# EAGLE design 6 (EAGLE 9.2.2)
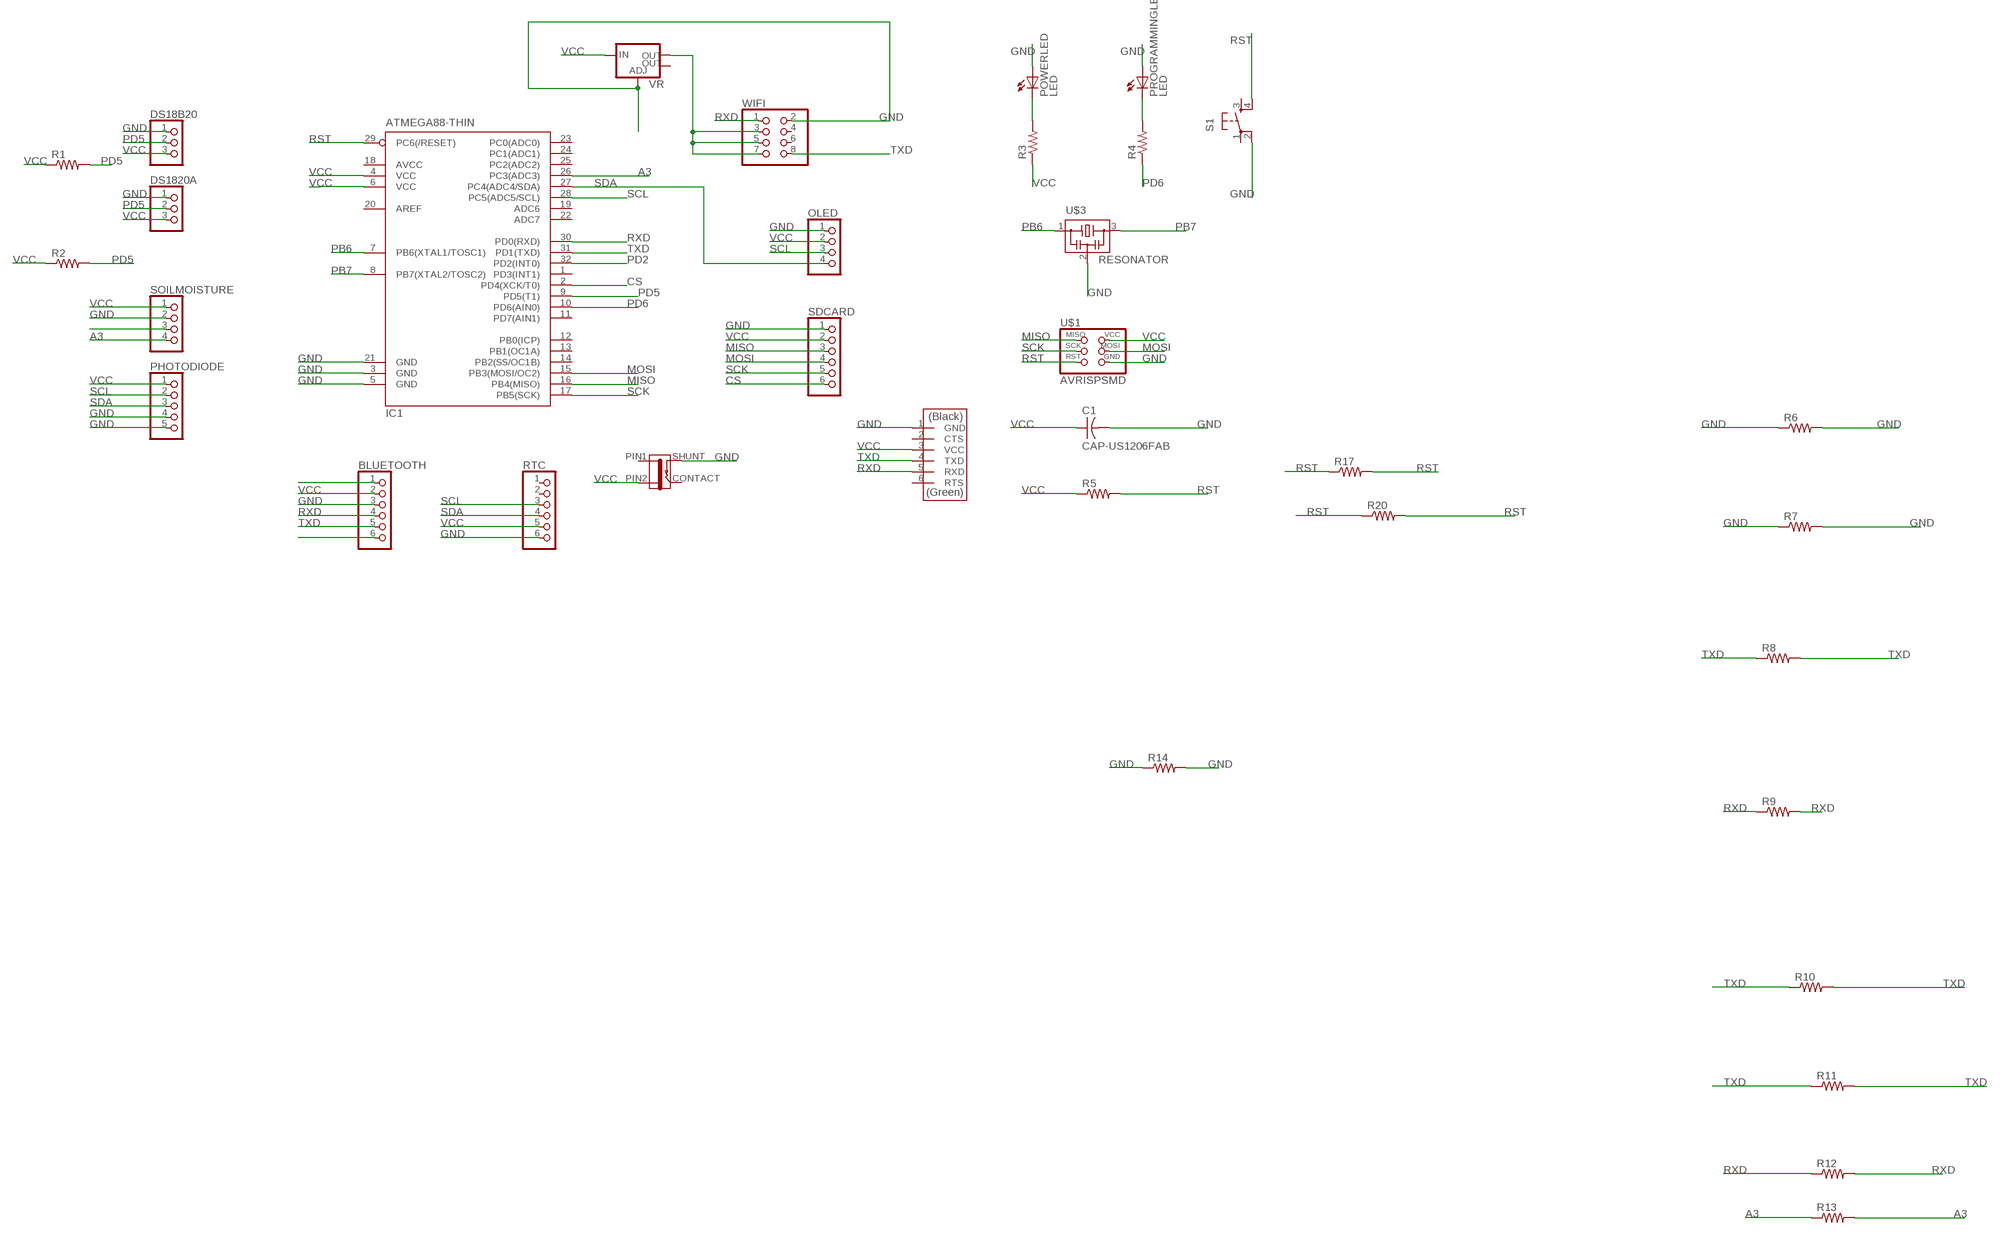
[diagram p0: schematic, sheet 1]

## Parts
BLUETOOTH  PINHD-1X6  [1X06]
C1  CAP-US1206FAB  [C1206FAB]
DS18B20  PINHD-1X3  [1X03]
DS1820A  PINHD-1X3  [1X03]
FTDI  FTDI-SMD-HEADER  [1X06SMD]
IC1  ATMEGA88-THIN  [TQFP32-08THIN]
J1  JACK-2.1MM  [PJ-002AH-SMT]
OLED  PINHD-1X4  [1X04]
PHOTODIODE  PINHD-1X5  [1X05]
POWERLED  LED  [LED1206]
PROGRAMMINGLED  LED  [LED1206]
R1  RES-US1206FAB  [R1206FAB]
R2  RES-US1206FAB  [R1206FAB]
R3  RES-US1206FAB  [R1206FAB]
R4  RES-US1206FAB  [R1206FAB]
R5  RES-US1206FAB  [R1206FAB]
R6  RES-US1206FAB  [R1206FAB]
R7  RES-US1206FAB  [R1206FAB]
R8  RES-US1206FAB  [R1206FAB]
R9  RES-US1206FAB  [R1206FAB]
R10  RES-US1206FAB  [R1206FAB]
R11  RES-US1206FAB  [R1206FAB]
R12  RES-US1206FAB  [R1206FAB]
R13  RES-US1206FAB  [R1206FAB]
R14  RES-US1206FAB  [R1206FAB]
R17  RES-US1206FAB  [R1206FAB]
R20  RES-US1206FAB  [R1206FAB]
RTC  PINHD-1X6  [1X06]
S1  6MM_SWITCH6MM_SWITCH  [6MM_SWITCH]
SDCARD  PINHD-1X6  [1X06]
SOILMOISTURE  PINHD-1X4  [1X04]
U$1  AVRISPSMD  [2X03SMD]
U$3  RESONATOR  [EFOBM]
VR  V_REG_LM1117SOT223  [SOT223]
WIFI  PINHD-2X4  [2X04]

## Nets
A3: IC1.26(PC3(ADC3)) R13.1 R13.2 SOILMOISTURE.4
CS: IC1.2(PD4(XCK/T0)) SDCARD.6
GND: BLUETOOTH.3 C1.2 DS18B20.1 DS1820A.1 FTDI.1(GND) IC1.3(GND) IC1.5(GND) IC1.21(GND) J1.SHUNT OLED.1 PHOTODIODE.4 PHOTODIODE.5 POWERLED.1(A) PROGRAMMINGLED.1(A) R6.1 R6.2 R7.1 R7.2 R14.1 R14.2 RTC.6 S1.2(P1) SDCARD.1 SOILMOISTURE.2 U$1.6(GND) U$3.2 VR.1(ADJ) WIFI.2
MISO: IC1.16(PB4(MISO)) SDCARD.3 U$1.1(MISO)
MOSI: IC1.15(PB3(MOSI/OC2)) SDCARD.4 U$1.4(MOSI)
N$1: BLUETOOTH.1
N$2: VR.2(OUT) WIFI.3 WIFI.5 WIFI.7
N$4: SOILMOISTURE.3
N$6: POWERLED.2(C) R3.2
N$8: BLUETOOTH.6
N$10: PROGRAMMINGLED.2(C) R4.2
PB6: IC1.7(PB6(XTAL1/TOSC1)) U$3.1
PB7: IC1.8(PB7(XTAL2/TOSC2)) U$3.3
PD2: IC1.32(PD2(INT0))
PD5: DS18B20.2 DS1820A.2 IC1.9(PD5(T1)) R1.2 R2.2
PD6: IC1.10(PD6(AIN0)) R4.1
RST: IC1.29(PC6(/RESET)) R5.2 R17.1 R17.2 R20.1 R20.2 S1.4(S1) U$1.5(RST)
RXD: BLUETOOTH.4 FTDI.5(RXD) IC1.30(PD0(RXD)) R9.1 R9.2 R12.1 R12.2 WIFI.1
SCK: IC1.17(PB5(SCK)) SDCARD.5 U$1.3(SCK)
SCL: IC1.28(PC5(ADC5/SCL)) OLED.3 PHOTODIODE.2 RTC.3
SDA: IC1.27(PC4(ADC4/SDA)) OLED.4 PHOTODIODE.3 RTC.4
TXD: BLUETOOTH.5 FTDI.4(TXD) IC1.31(PD1(TXD)) R8.1 R8.2 R10.1 R10.2 R11.1 R11.2 WIFI.8
VCC: BLUETOOTH.2 C1.1 DS18B20.3 DS1820A.3 FTDI.3(VCC) IC1.4(VCC) IC1.6(VCC) J1.PIN2 OLED.2 PHOTODIODE.1 R1.1 R2.1 R3.1 R5.1 RTC.5 SDCARD.2 SOILMOISTURE.1 U$1.2(VCC) VR.3(IN)
Unconnected: FTDI.2(CTS) FTDI.6(RTS) IC1.1(PD3(INT1)) IC1.11(PD7(AIN1)) IC1.12(PB0(ICP)) IC1.13(PB1(OC1A)) IC1.14(PB2(SS/OC1B)) IC1.19(ADC6) IC1.20(AREF) IC1.22(ADC7) IC1.23(PC0(ADC0)) IC1.24(PC1(ADC1)) IC1.25(PC2(ADC2)) RTC.1 RTC.2 S1.1(P) S1.3(S) VR.4(OUT) WIFI.4 WIFI.6

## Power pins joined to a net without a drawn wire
AVCC: IC1.18(AVCC)
CONTACT: J1.CONTACT
PIN1: J1.PIN1

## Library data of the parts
BLUETOOTH RTC SDCARD = pinhead:PINHD-1X6: PIN HEADER
C1 = fab:CAP-US
DS18B20 DS1820A = pinhead:PINHD-1X3: PIN HEADER
FTDI = fab:FTDI-SMD-HEADER
IC1 = fab:ATMEGA88-THIN
J1 = fab:JACK-2.1MM: SMD DC power jack PJ-002AH-SMT As found in the fablab inventory. Made by Zaerc.
OLED SOILMOISTURE = pinhead:PINHD-1X4: PIN HEADER
PHOTODIODE = pinhead:PINHD-1X5: PIN HEADER
POWERLED PROGRAMMINGLED = fab:LED: LED
R1-R14 R17 R20 = fab:RES-US: Resistor (US Symbol)
S1 = fab:6MM_SWITCH: OMRON SWITCH
U$1 = fab:AVRISP
U$3 = fab:RESONATOR
VR = fab:V_REG_LM1117: Voltage Regulator LM1117 Standard adjustable voltage regulator but in SMD form. Spark Fun Electronics SKU : COM-00595; PROD_ID: VREG-08170
WIFI = pinhead:PINHD-2X4: PIN HEADER

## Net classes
0 default: width 0.152 mm, clearance 0.4 mm

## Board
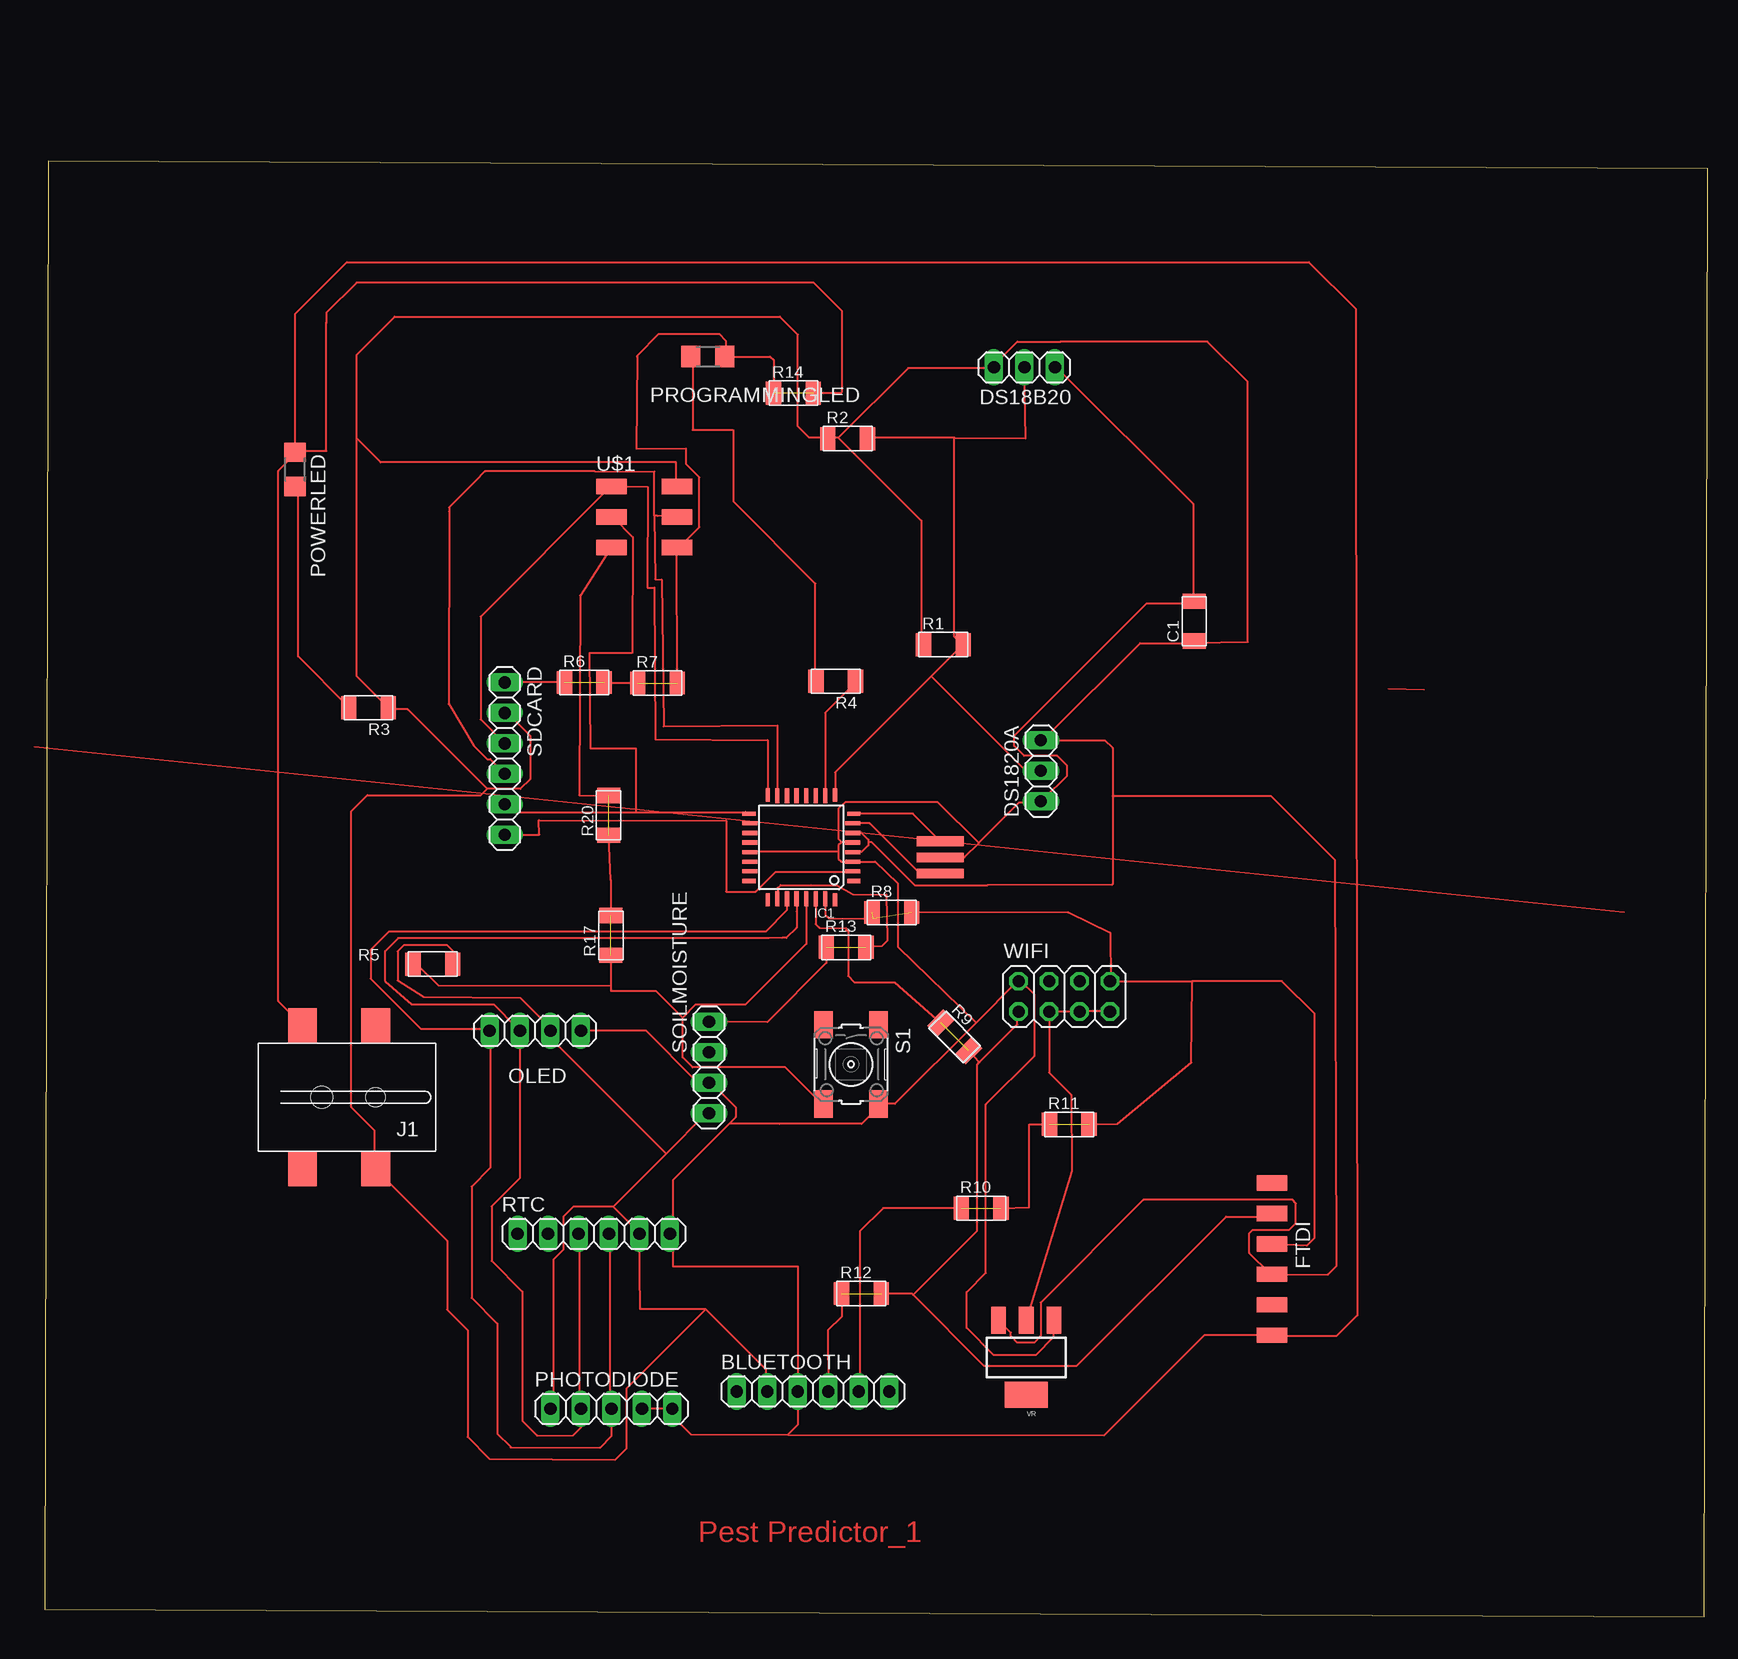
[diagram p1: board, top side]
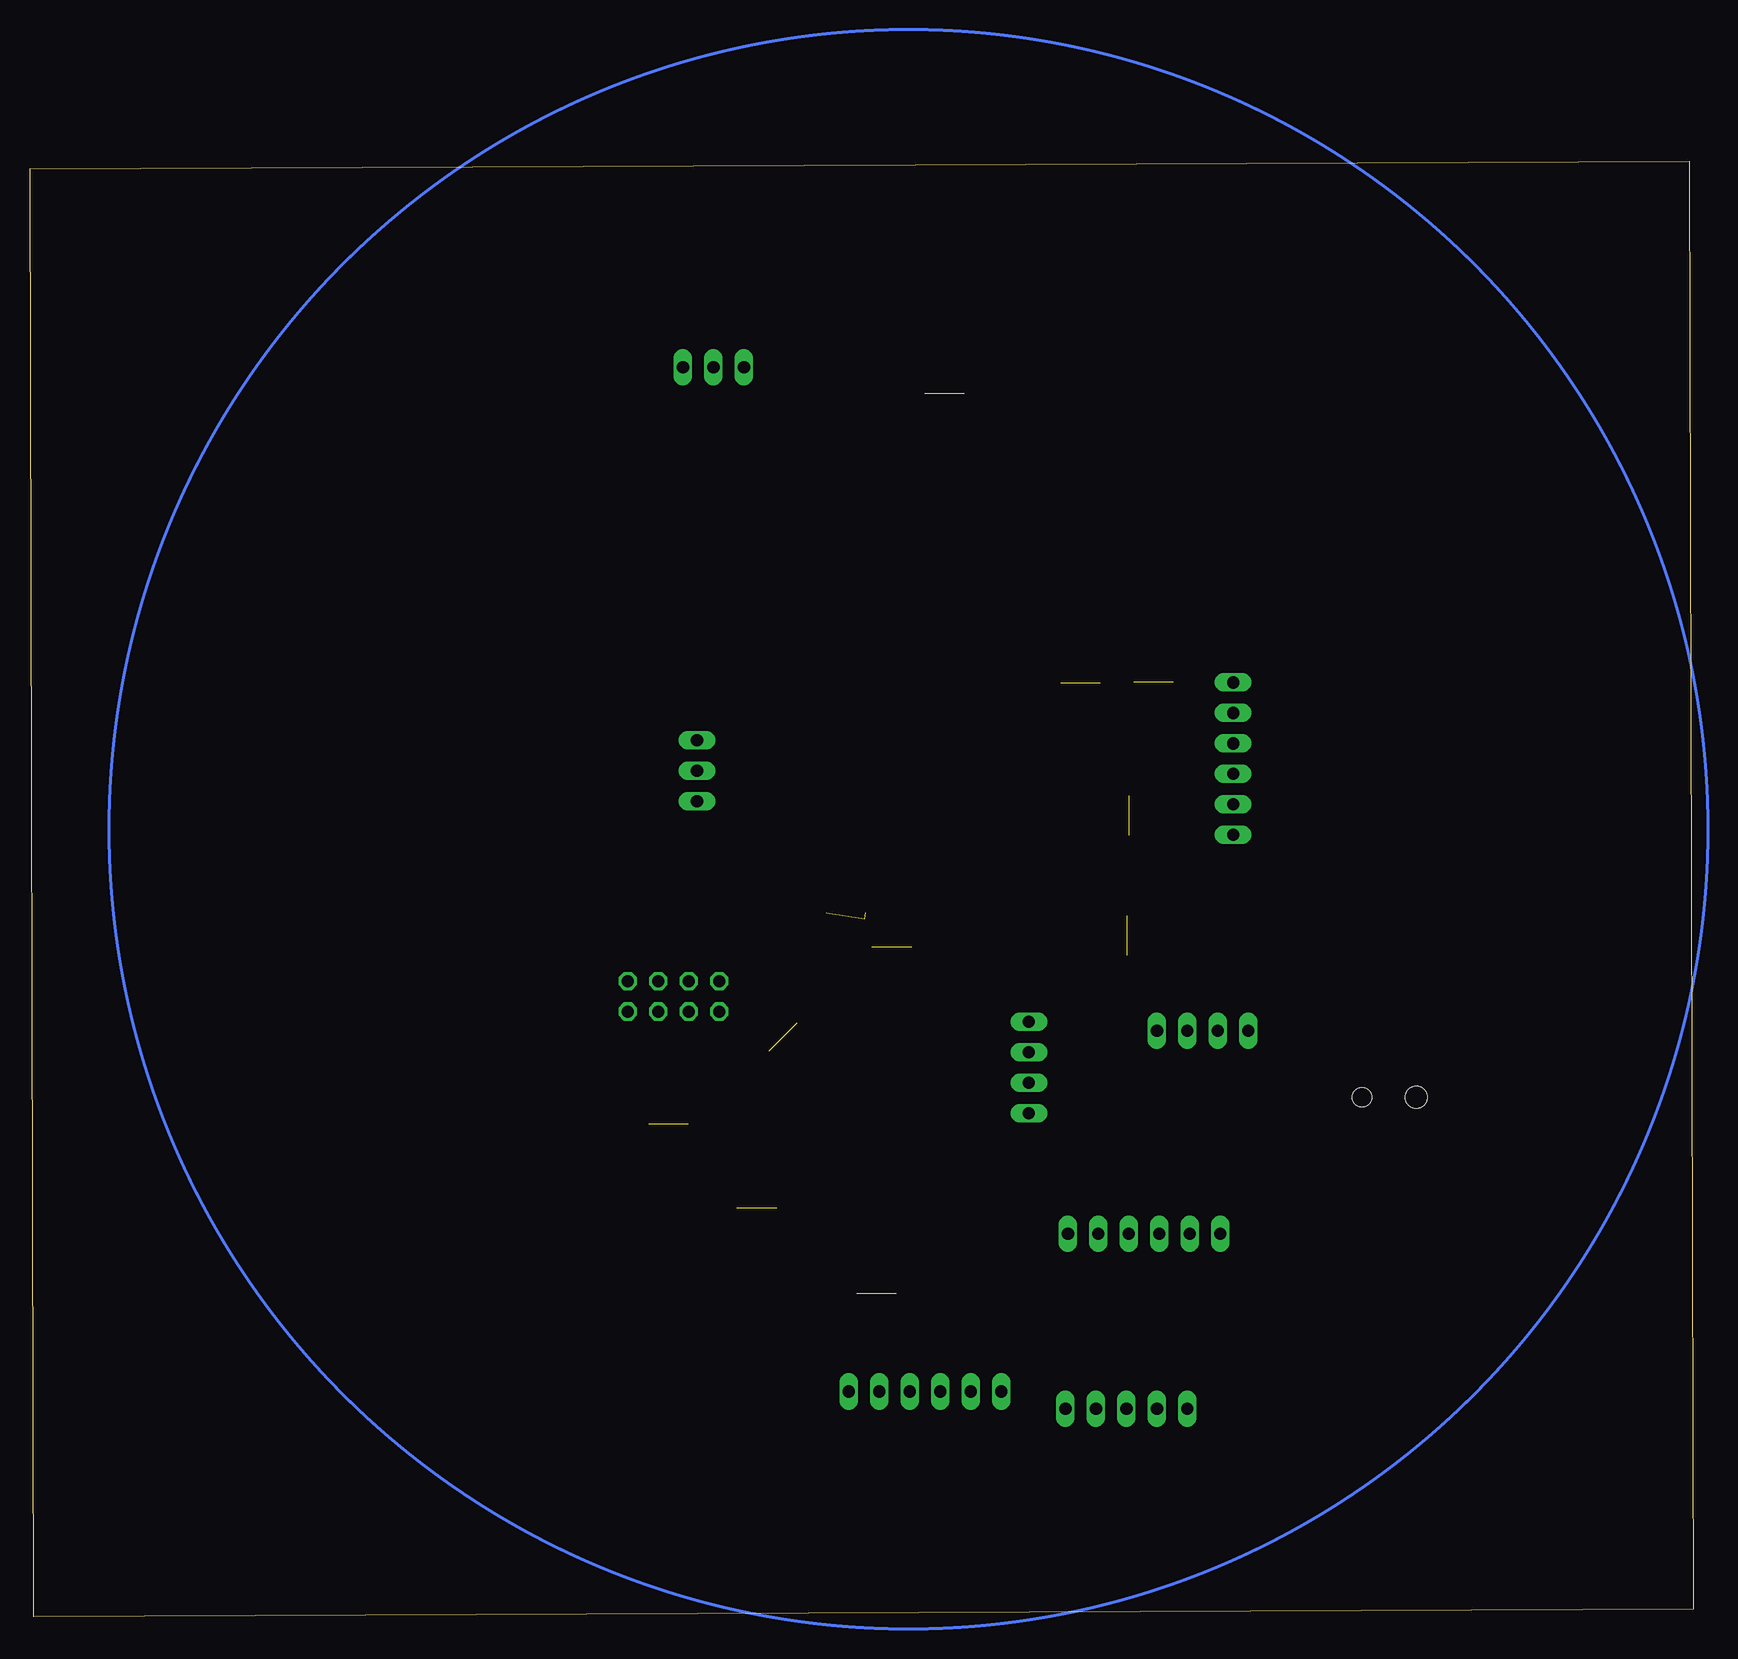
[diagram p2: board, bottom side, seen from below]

Size 138.59 x 121.29 mm. Coordinates in mm from the lower left corner, seen from the top.
Outline: 0,0.61 138.28,0 138.59,120.68 0.3,121.29 0,0.61
Copper layers (1*16): Top 0.035mm / dielectric 1.5mm / Bottom 0.035mm
Design rules "default *": minimum track width 6mil, minimum drill 0.35mm, track to track 0.4mm, track to pad 6mil, pad to pad 6mil, via to via 6mil, smd to smd 6mil, copper to edge 40mil, drill to drill 6mil, minimum pad ring 10mil, minimum via ring 8mil, stop-mask expansion 4mil, vias tented up to drill 0mil, thermal gap 10mil

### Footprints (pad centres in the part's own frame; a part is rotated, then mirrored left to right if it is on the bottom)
1X06 = drill 1.016 long: 1 -6.35,0; 2 -3.81,0; 3 -1.27,0; 4 1.27,0; 5 3.81,0; 6 6.35,0
C1206FAB = smd 1.27 x 1.905: 1 -1.651,0; 2 1.651,0
1X03 = drill 1.016 long: 1 -2.54,0; 2 0,0; 3 2.54,0
1X06SMD = smd 2.54 x 1.27: 1 0,6.35; 2 0,3.81; 3 0,1.27; 4 0,-1.27; 5 0,-3.81; 6 0,-6.35
TQFP32-08THIN = smd 1.118 x 0.356: 1 -4.369,2.8; 8 -4.369,-2.8; 17 4.369,-2.8; 24 4.369,2.8 | smd 1.27 x 0.356: 2 -4.293,2; 3 -4.293,1.2; 4 -4.293,0.4; 5 -4.293,-0.4; 6 -4.293,-1.2; 7 -4.293,-2; 18 4.293,-2; 19 4.293,-1.2; 20 4.293,-0.4; 21 4.293,0.4; 22 4.293,1.2; 23 4.293,2 | smd 0.356 x 1.118: 9 -2.8,-4.369; 16 2.8,-4.369; 25 2.8,4.369; 32 -2.8,4.369 | smd 0.356 x 1.27: 10 -2,-4.293; 14 1.2,-4.293; 15 2,-4.293; 26 2,4.293; 27 1.2,4.293; 31 -2,4.293 | smd 0.35 x 1.27: 11 -1.2,-4.293; 12 -0.4,-4.293; 13 0.4,-4.293; 28 0.4,4.293; 29 -0.4,4.293; 30 -1.2,4.293
PJ-002AH-SMT = smd 2.4 x 2.8: CONTACT -2.4,-6; PIN1 3.7,6; PIN2 -2.4,6; SHUNT 3.7,-6 | hole 1.6: -2.4,0 | hole 1.8: 2.1,0
1X04 = drill 1.016 long: 1 -3.81,0; 2 -1.27,0; 3 1.27,0; 4 3.81,0
1X05 = drill 1.016 long: 1 -5.08,0; 2 -2.54,0; 3 0,0; 4 2.54,0; 5 5.08,0
LED1206 = smd 1.6 x 1.803: 1 -1.422,0; 2 1.422,0
R1206FAB = smd 1.27 x 1.905: 1 -1.651,0; 2 1.651,0
6MM_SWITCH = smd 2.286 x 1.524: 1 -3.302,2.286; 2 3.302,2.286; 3 -3.302,-2.286; 4 3.302,-2.286
2X03SMD = smd 2.54 x 1.27: 1 -2.54,2.54; 2 2.92,2.54; 3 -2.54,0; 4 2.92,0; 5 -2.54,-2.54; 6 2.92,-2.54
EFOBM = smd 0.8 x 3.9: 1 -1.35,0; 2 0,0; 3 1.35,0
SOT223 = smd 1.219 x 2.235: 1 -2.311,-3.099; 2 0,-3.099; 3 2.311,-3.099 | smd 3.6 x 2.2: 4 0,3.099
2X04 = drill 1.016 octagon: 1 -3.81,-1.27; 2 -3.81,1.27; 3 -1.27,-1.27; 4 -1.27,1.27; 5 1.27,-1.27; 6 1.27,1.27; 7 3.81,-1.27; 8 3.81,1.27

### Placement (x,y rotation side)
BLUETOOTH  64.01,18.77 0 top
C1  95.78,82.96 90 top
DS18B20  81.64,104.11 180 top
DS1820A  83.01,70.48 90 top
FTDI  102.29,29.79 180 top
IC1  63.04,64.11 180 top
J1  25.17,43.28 180 top
OLED  40.87,48.82 180 top
PHOTODIODE  47.22,17.32 0 top
POWERLED  20.85,95.61 270 top
PROGRAMMINGLED  55.24,105 180 top
R1  74.88,81 0 top
R2  66.9,98.17 0 top
R3  26.97,75.74 180 top
R4  65.91,77.95 180 top
R5  32.33,54.38 180 top
R6  44.96,77.85 0 top
R7  51.05,77.8 0 top
R8  70.59,58.67 0 top
R9  75.82,48.31 315 top
R10  78.03,34.04 0 top
R11  85.37,41.02 0 top
R12  68.05,26.92 0 top
R13  66.78,55.78 0 top
R14  62.38,101.96 0 top
R17  47.17,56.77 90 top
R20  46.99,66.78 90 top
RTC  45.75,31.9 0 top
S1  67.18,46.02 270 top
SDCARD  38.33,71.5 270 top
SOILMOISTURE  55.35,45.77 90 top
U$1  49.76,91.64 0 top
U$3  74.63,63.27 90 top
VR  81.79,21.59 180 top
WIFI  84.96,51.69 0 top

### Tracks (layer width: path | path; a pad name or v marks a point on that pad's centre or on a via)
A3  (1 unrouted)
  Top 0.152: IC1.26 61.07,59.83 61.07,60.71 61.32,60.96 63.83,60.96 65.99,60.96 67.34,60.2 70.13,60.17 70.22,56.46 70.22,56.34 69.75,55.87 R13.2 | SOILMOISTURE.4 60.2,49.55 65.13,54.48 R13.1
CS
  Top 0.152: IC1.2 67.24,62.07 60.89,62.07 59.24,60.41 56.77,60.41 56.77,66.35 41.17,66.37 41.22,65.18 SDCARD.6
GND  (3 unrouted)
  Top 0.152: DS18B20.1 84.37,104.05 95.69,92.73 95.69,84.72 C1.2 95.69,84.44 91.83,84.44 80.78,73.39 80.78,72.56 81.61,71.73 84.37,71.73 85.2,70.91 85.2,70.08 83.26,68.14 DS1820A.1 82.99,67.87 81.21,67.87 77.82,64.48 | 66.14,63.72 66.14,64.28 66.42,64.55 | 66.14,63.72 66.14,63.17 66.42,62.9 67.24,62.9 IC1.3 | 66.42,64.55 67.24,64.55 IC1.5 | 66.14,63.72 58.96,63.72 IC1.21 | U$3.2 76.64,63.27 77.83,64.46 77.82,64.48 | 66.42,64.55 66.14,64.83 66.14,67.31 66.69,67.87 74.43,67.87 77.82,64.48 | 57.02,41.07 57.58,41.63 57.58,42.46 55.37,44.67 SOILMOISTURE.2 55.09,44.67 54.26,44.67 50.12,48.81 44.87,48.81 OLED.1 | 57.02,41.07 52.33,36.38 52.33,31.96 RTC.6 52.33,31.69 52.33,29.2 62.76,29.18 BLUETOOTH.3 62.74,15.99 61.92,15.18 | VR.1 84.09,24.5 84.09,23.32 82.56,21.79 79.09,21.79 76.81,24.07 76.81,27.04 78.42,28.65 78.42,42.7 82.44,46.71 82.44,51.85 81.33,52.95 WIFI.2 81.05,52.95 77.61,49.51 | 77.61,49.51 70.84,42.73 69.73,42.73 S1.2 69.45,42.46 68.07,41.08 61.21,41.08 61.22,41.07 57.02,41.07 | 67.52,62.9 IC1.3 | POWERLED.1 20.84,96.87 19.46,95.49 19.46,51.3 21.4,49.36 J1.SHUNT | PHOTODIODE.4 49.84,17.32 52.05,17.32 PHOTODIODE.5 | 102.05,23.4 FTDI.1 | 52.33,17.32 PHOTODIODE.5 | POWERLED.1 21.12,97.14 23.47,97.14 23.47,107.82 23.47,107.87 23.47,108.66 25.98,111.18 64.06,111.18 66.4,108.84 66.4,102.03 66.32,101.96 R14.2 | 102.32,23.4 FTDI.1 | 56.47,105.15 PROGRAMMINGLED.1 | R6.1 SDCARD.1 | R7.1 46.68,77.78 R6.2 | R7.2 U$1.6 52.69,89.11 52.8,89.12 52.88,89.13 54.54,90.79 54.54,94.93 53.43,96.04 53.43,97.36 49.3,97.33 49.36,104.95 49.36,105.08 51.18,106.89 56.18,106.89 56.74,106.34 56.74,105.06 56.8,105 PROGRAMMINGLED.1
  Top 0.152: IC1.3 69.19,62.92 71.09,61.11 71.09,55.83 77.61,49.51 | 61.92,15.18 53.85,15.19 52.3,16.74 PHOTODIODE.5 | 61.92,15.18 88.29,15.13 96.6,23.44 FTDI.1 | FTDI.1 102.34,23.39 107.65,23.39 109.35,25.1 109.39,25.1 109.28,101.14 109.28,108.93 105.33,112.88 25.17,112.88 20.85,108.56 POWERLED.1 | PROGRAMMINGLED.1 60.45,105 60.73,104.72 R14.1
MISO
  Top 0.152: IC1.16 60.24,73.05 50.88,73.1 50.8,85.75 50.22,85.75 50.24,94.16 U$1.1 47.08,94.11 36.31,83.33 36.31,74.77 38.24,72.84 SDCARD.3
MOSI
  Top 0.152: IC1.15 61.04,74.27 51.56,74.19 51.41,86.41 50.85,86.46 50.8,91.75 | SDCARD.4 38.24,70.35 37.14,71.46 36.86,71.46 35.76,72.56 33.65,76.07 33.7,92.1 33.7,92.45 35.91,94.67 36.68,95.43 45.85,95.44 50.8,95.43 50.8,91.75 | U$1.4 51.05,91.73 50.8,91.75
N$2
  Top 0.152: WIFI.7 88.51,50.47 86.3,50.47 WIFI.5 86.03,50.47 83.82,50.47 WIFI.3 83.69,45.33 85.56,43.46 85.52,43.46 85.58,37.14 VR.2
N$6
  Top 0.152: POWERLED.2 21.12,94.11 21.12,80.02 25.26,75.88 R3.2
N$10
  Top 0.152: PROGRAMMINGLED.2 53.99,104.88 53.99,98.91 57.35,98.91 57.37,92.93 64.21,86.1 64.21,78.09 R4.2
PB6
  Top 0.152: IC1.7 68.73,66.11 72.77,62.07 74.43,62.07 U$3.1
PB7
  Top 0.152: IC1.8 72.34,66.91 74.43,64.83 U$3.3
PD5
  Top 0.152: 75.81,98.25 68.63,98.25 R2.2 | 73.87,78.36 76.36,80.85 R1.2 76.36,81.12 75.81,81.68 75.81,98.25 | 73.87,78.36 65.86,70.35 65.86,68.7 IC1.9 | 73.87,78.36 81.61,70.63 82.99,70.63 DS1820A.2 | 75.81,98.25 81.74,98.2 DS18B20.2
PD6
  Top 0.152: IC1.10 65.04,68.42 65.04,75.32 67.52,77.81 R4.1
RST  (2 unrouted)
  Top 0.152: IC1.29 63.45,56.07 58.41,51.02 54.26,51.02 53.16,49.91 | 53.16,49.91 53.16,46.6 53.99,45.77 61.72,45.77 64.76,42.73 S1.4 | 53.16,49.91 50.95,52.12 47.17,52.12 47.17,52.58 | R5.2 30.79,54.33 31.06,54.33 32.79,52.6 47.17,52.58 | 47.34,88.98 U$1.5 44.6,85.08 44.52,68.45 R20.2 | R17.2 47.17,61.38 R20.1 | R17.1 47.17,52.58
RXD  (2 unrouted)
  Top 0.152: FTDI.5 102.05,33.34 98.44,33.34 86.01,20.91 78.26,20.91 72.36,26.81 | 77.89,46.19 77.69,46 77.69,32.15 72.36,26.81 | 77.89,46.19 81.05,49.36 81.05,50.19 WIFI.1 | 77.89,46.19 R9.2 | BLUETOOTH.4 65.26,23.85 66.4,24.98 R12.1 | R9.1 70.82,52.86 67.47,52.86 66.93,53.4 66.93,57.08 66.78,57.23 66.78,57.38 64.57,57.42 64.52,57.42 64.24,57.71 IC1.30 | 72.36,26.81 72.25,26.92 R12.2
SCK
  Top 0.152: 49.25,67.04 39.07,67.04 38.52,67.59 SDCARD.5 | 49.25,67.04 58.41,67.04 IC1.17 | U$1.3 47.36,91.62 49.02,89.96 48.95,80.29 45.39,80.29 45.47,72.36 49.25,72.36 49.25,67.04
SCL
  Top 0.152: RTC.3 44.6,31.69 44.6,17.6 PHOTODIODE.2 44.68,15.76 44.03,15.11 41.04,15.09 39.8,16.33 39.8,27.08 37.24,29.64 37.24,34.19 39.6,36.55 OLED.3 39.35,49.09 37.42,51.02 30.59,51.02 28.37,52.94 28.35,55.46 29.44,56.54 60.34,56.54 61.44,56.57 61.8,56.57 62.66,57.43 62.65,58.78 IC1.28
SDA
  Top 0.152: RTC.4 47.08,31.69 47.08,17.6 PHOTODIODE.3 47.22,15.04 46.28,14.1 38.81,14.11 38.81,14.15 37.72,15.24 37.72,24.41 35.56,26.57 35.56,35.84 37.14,37.42 37.14,48.81 OLED.4 36.93,49 31.31,49 27.15,53.16 27.15,55.57 28.68,57.1 60.06,57.1 61.85,58.88 IC1.27
TXD  (4 unrouted)
  Top 0.152: 103.43,31.13 102.32,31.13 FTDI.4 105.16,30.94 105.18,30.94 105.82,31.57 105.82,50.24 103.1,52.96 95.61,52.96 | R8.2 85.28,58.69 88.77,57 88.83,52.91 88.79,52.95 WIFI.8 95.61,52.96 | R10.2 82.02,34.11 82.04,41.02 R11.1 | R11.2 89.36,41.07 95.55,46.19 95.61,52.96 | IC1.31 65.05,58.5 65.35,58.19 65.38,58.19 69.04,58.17 | BLUETOOTH.5 67.92,18.87 | 67.92,18.87 68.51,19.46 | R10.1 69.85,34.04 67.92,32.11 67.92,18.87
VCC
  Top 0.152: VR.3 79.67,24.5 80.5,23.68 80.5,23.4 81.05,22.85 82.44,22.85 82.99,23.4 82.99,26.16 91.55,34.72 103.98,34.72 104.26,34.45 104.26,32.79 103.7,32.24 100.67,32.24 100.39,31.96 100.39,30.3 102.05,28.65 FTDI.3 106.91,28.5 107.64,29.24 107.64,29.52 107.52,63.04 102.19,68.38 88.98,68.38 | 68.63,64.53 68.63,64.75 68.05,65.33 67.39,65.33 IC1.6 | 68.63,64.53 68.63,64.28 68.07,63.72 67.52,63.72 IC1.4 | 95.69,81.12 91.27,81.12 83.54,73.39 | 83.54,73.39 83.26,73.12 DS1820A.3 | 95.69,81.12 C1.1 | 68.63,64.53 68.92,64.53 72.49,60.96 78.57,60.96 88.93,60.99 88.98,61.04 88.98,68.38 | 83.54,73.39 DS1820A.3 | 47.36,34.17 44.04,34.17 43.22,33.34 43.22,30.58 42.39,29.75 42.39,17.6 PHOTODIODE.1 | 47.36,34.17 49.57,31.96 RTC.5 49.61,25.63 55.09,25.61 | 47.36,34.17 51.78,38.59 | 51.78,38.59 55.09,41.9 SOILMOISTURE.1 | 55.09,25.61 60.06,20.64 60.06,18.98 BLUETOOTH.2 | 51.78,38.59 42.39,47.98 42.39,48.81 OLED.2 42.11,49.09 39.62,51.57 31.57,51.64 29.41,53.02 29.41,55.44 29.96,55.99 31.34,55.99 arc90 31.35,55.98 33.5,55.98 33.99,55.5 R5.1 | 36.86,68.97 30.23,75.6 28.85,75.6 R3.1 25.98,78.38 25.98,98.2 | 36.86,68.97 39.62,68.97 40.45,69.8 40.45,73.39 38.52,75.32 SDCARD.2 | 66.14,98.25 65.31,98.25 R2.1 65.18,98.25 63.7,98.25 62.76,99.19 62.76,106.83 61.26,108.33 29.16,108.33 25.98,105.16 25.98,98.2 | 66.14,98.25 71.94,104.05 78.85,104.05 DS18B20.3 79.12,104.33 81.05,106.26 84.65,106.26 96.88,106.25 100.23,102.89 100.23,101.55 100.25,81.2 95.69,81.12 | 66.14,98.25 73.05,91.34 73.05,81.12 R1.1 | U$1.2 52.61,94.38 52.61,96.19 27.99,96.19 25.98,98.2 | 55.09,25.61 48.46,18.98 48.46,15.94 48.46,14.25 48.46,14 47.52,13.06 37.06,13.15 35.23,14.98 35.23,23.88 33.53,25.58 33.53,31.33 J1.PIN2 27.47,37.49 27.47,40.52 25.54,42.46 25.54,67.12 26.87,68.45 36.34,68.45 36.86,68.97
  Top 0.152: DS1820A.3 88.34,73.03 88.98,72.39 88.98,68.38
(copper drawn outside any net)
  shapes: Bottom circle x1, Top area x2

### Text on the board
Top: Pest Predictor_1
